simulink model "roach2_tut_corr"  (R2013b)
settings: Solver=VariableStepDiscrete  SolverMode=SingleTasking  StartTime=0.0  StopTime=100  RelTol=1e-3
undefined symbols (not defined in the file): add_latency, addr_width, Bit, bitfield, BitWidth, bram_latency, burst_size, casper_library_scopes, conv_latency, data_width, DelayLen, fan_latency, FFTSize, FFTStage, getfield, increment, led, Location, Lower, mult_latency, mux_latency, n_bits, n_bits_data, n_inputs, n_streams, n_taps, neg_latency, negate_latency, nsamples, pfb_size, pulse_len, reset_period, ROACH, ROACH2, snapshot, sx475t, sync_period, sync_period_bits, Upper, UseCounter, Width
libraries: xbsIndex_r4 x24444, casper_library_misc x73, xbsReplacements_r4 x34, casper_library_delays x14, xps_library x7
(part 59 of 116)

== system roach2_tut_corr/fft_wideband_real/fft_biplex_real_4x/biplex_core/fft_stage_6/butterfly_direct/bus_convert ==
  din : Inport
  bussify : Subsystem  AncestorBlock=casper_library_flow_control/bus_create
  conv1 : Subsystem  AncestorBlock=casper_library_misc/convert_of
  conv10 : Subsystem  AncestorBlock=casper_library_misc/convert_of
  conv11 : Subsystem  AncestorBlock=casper_library_misc/convert_of
  conv12 : Subsystem  AncestorBlock=casper_library_misc/convert_of
  conv13 : Subsystem  AncestorBlock=casper_library_misc/convert_of
  conv14 : Subsystem  AncestorBlock=casper_library_misc/convert_of
  conv15 : Subsystem  AncestorBlock=casper_library_misc/convert_of
  conv16 : Subsystem  AncestorBlock=casper_library_misc/convert_of
  conv2 : Subsystem  AncestorBlock=casper_library_misc/convert_of
  conv3 : Subsystem  AncestorBlock=casper_library_misc/convert_of
  conv4 : Subsystem  AncestorBlock=casper_library_misc/convert_of
  conv5 : Subsystem  AncestorBlock=casper_library_misc/convert_of
  conv6 : Subsystem  AncestorBlock=casper_library_misc/convert_of
  conv7 : Subsystem  AncestorBlock=casper_library_misc/convert_of
  conv8 : Subsystem  AncestorBlock=casper_library_misc/convert_of
  conv9 : Subsystem  AncestorBlock=casper_library_misc/convert_of
  debus : Subsystem  AncestorBlock=casper_library_flow_control/bus_expand
  of_bussify : Subsystem  AncestorBlock=casper_library_flow_control/bus_create
  dout : Outport
  overflow : Outport  Port=2
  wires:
  din/1 -> debus/1(bus_in)
  debus/1(msb_out16) -> conv1/1(din)
  debus/2(out15) -> conv2/1(din)
  debus/3(out14) -> conv3/1(din)
  debus/4(out13) -> conv4/1(din)
  debus/5(out12) -> conv5/1(din)
  debus/6(out11) -> conv6/1(din)
  debus/7(out10) -> conv7/1(din)
  debus/8(out9) -> conv8/1(din)
  debus/9(out8) -> conv9/1(din)
  debus/10(out7) -> conv10/1(din)
  debus/11(out6) -> conv11/1(din)
  debus/12(out5) -> conv12/1(din)
  debus/13(out4) -> conv13/1(din)
  debus/14(out3) -> conv14/1(din)
  debus/15(out2) -> conv15/1(din)
  debus/16(lsb_out1) -> conv16/1(din)
  conv1/1(dout) -> bussify/1(in1)
  conv2/1(dout) -> bussify/2(in2)
  conv3/1(dout) -> bussify/3(in3)
  conv4/1(dout) -> bussify/4(in4)
  conv5/1(dout) -> bussify/5(in5)
  conv6/1(dout) -> bussify/6(in6)
  conv7/1(dout) -> bussify/7(in7)
  conv8/1(dout) -> bussify/8(in8)
  conv9/1(dout) -> bussify/9(in9)
  conv10/1(dout) -> bussify/10(in10)
  conv11/1(dout) -> bussify/11(in11)
  conv12/1(dout) -> bussify/12(in12)
  conv13/1(dout) -> bussify/13(in13)
  conv14/1(dout) -> bussify/14(in14)
  conv15/1(dout) -> bussify/15(in15)
  conv16/1(dout) -> bussify/16(in16)
  conv1/2(of) -> of_bussify/1(in1)
  conv2/2(of) -> of_bussify/2(in2)
  conv3/2(of) -> of_bussify/3(in3)
  conv4/2(of) -> of_bussify/4(in4)
  conv5/2(of) -> of_bussify/5(in5)
  conv6/2(of) -> of_bussify/6(in6)
  conv7/2(of) -> of_bussify/7(in7)
  conv8/2(of) -> of_bussify/8(in8)
  conv9/2(of) -> of_bussify/9(in9)
  conv10/2(of) -> of_bussify/10(in10)
  conv11/2(of) -> of_bussify/11(in11)
  conv12/2(of) -> of_bussify/12(in12)
  conv13/2(of) -> of_bussify/13(in13)
  conv14/2(of) -> of_bussify/14(in14)
  conv15/2(of) -> of_bussify/15(in15)
  conv16/2(of) -> of_bussify/16(in16)
  bussify/1(bus_out) -> dout/1
  of_bussify/1(bus_out) -> overflow/1

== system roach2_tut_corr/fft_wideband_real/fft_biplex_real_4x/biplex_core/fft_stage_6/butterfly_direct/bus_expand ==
  bus_in : Inport
  reinterpret1 : xbsIndex_r4/Reinterpret  force_arith_type=on  arith_type=Unsigned  force_bin_pt=on  bin_pt=0  block_type=reinterpret
  reinterpret2 : xbsIndex_r4/Reinterpret  force_arith_type=on  arith_type=Unsigned  force_bin_pt=on  bin_pt=0  block_type=reinterpret
  slice1 : xbsIndex_r4/Slice  nbits=144  boolean_output=off  mode=Upper Bit Location + Width  bit1=-144  base1=MSB of Input  bit0=0  base0=LSB of Input  dbl_ovrd=off  block_type=slice
  slice2 : xbsIndex_r4/Slice  nbits=144  boolean_output=off  mode=Upper Bit Location + Width  bit1=0  base1=MSB of Input  bit0=0  base0=LSB of Input  dbl_ovrd=off  block_type=slice
  msb_out2 : Outport
  lsb_out1 : Outport  Port=2
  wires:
  bus_in/1 -> slice2/1, slice1/1
  slice2/1 -> reinterpret2/1
  reinterpret2/1 -> msb_out2/1
  slice1/1 -> reinterpret1/1
  reinterpret1/1 -> lsb_out1/1

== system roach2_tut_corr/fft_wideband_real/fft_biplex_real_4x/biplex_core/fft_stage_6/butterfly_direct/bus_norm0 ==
  din : Inport
  bussify : Subsystem  AncestorBlock=casper_library_flow_control/bus_create
  conv{1..16} (16 alike) : xbsIndex_r4/Convert  gui_display_data_type=Fixed-point  arith_type="Signed  (2's comp)"  n_bits=21  bin_pt=18  float_type=Single  exp_bits=8  fraction_bits=24  quantization=Truncate  overflow=Wrap  en=off  latency=0  dbl_ovrd=off  pipeline=on  block_type=convert
  debus : Subsystem  AncestorBlock=casper_library_flow_control/bus_expand
  dout : Outport
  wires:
  din/1 -> debus/1(bus_in)
  debus/1(msb_out16) -> conv1/1
  debus/2(out15) -> conv2/1
  debus/3(out14) -> conv3/1
  debus/4(out13) -> conv4/1
  debus/5(out12) -> conv5/1
  debus/6(out11) -> conv6/1
  debus/7(out10) -> conv7/1
  debus/8(out9) -> conv8/1
  debus/9(out8) -> conv9/1
  debus/10(out7) -> conv10/1
  debus/11(out6) -> conv11/1
  debus/12(out5) -> conv12/1
  debus/13(out4) -> conv13/1
  debus/14(out3) -> conv14/1
  debus/15(out2) -> conv15/1
  debus/16(lsb_out1) -> conv16/1
  conv1/1 -> bussify/1(in1)
  conv2/1 -> bussify/2(in2)
  conv3/1 -> bussify/3(in3)
  conv4/1 -> bussify/4(in4)
  conv5/1 -> bussify/5(in5)
  conv6/1 -> bussify/6(in6)
  conv7/1 -> bussify/7(in7)
  conv8/1 -> bussify/8(in8)
  conv9/1 -> bussify/9(in9)
  conv10/1 -> bussify/10(in10)
  conv11/1 -> bussify/11(in11)
  conv12/1 -> bussify/12(in12)
  conv13/1 -> bussify/13(in13)
  conv14/1 -> bussify/14(in14)
  conv15/1 -> bussify/15(in15)
  conv16/1 -> bussify/16(in16)
  bussify/1(bus_out) -> dout/1

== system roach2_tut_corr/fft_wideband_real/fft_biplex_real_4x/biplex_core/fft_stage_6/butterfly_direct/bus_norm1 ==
  din : Inport
  bussify : Subsystem  AncestorBlock=casper_library_flow_control/bus_create
  conv1 : Subsystem  AncestorBlock=casper_library_misc/convert
  conv10 : Subsystem  AncestorBlock=casper_library_misc/convert
  conv11 : Subsystem  AncestorBlock=casper_library_misc/convert
  conv12 : Subsystem  AncestorBlock=casper_library_misc/convert
  conv13 : Subsystem  AncestorBlock=casper_library_misc/convert
  conv14 : Subsystem  AncestorBlock=casper_library_misc/convert
  conv15 : Subsystem  AncestorBlock=casper_library_misc/convert
  conv16 : Subsystem  AncestorBlock=casper_library_misc/convert
  conv2 : Subsystem  AncestorBlock=casper_library_misc/convert
  conv3 : Subsystem  AncestorBlock=casper_library_misc/convert
  conv4 : Subsystem  AncestorBlock=casper_library_misc/convert
  conv5 : Subsystem  AncestorBlock=casper_library_misc/convert
  conv6 : Subsystem  AncestorBlock=casper_library_misc/convert
  conv7 : Subsystem  AncestorBlock=casper_library_misc/convert
  conv8 : Subsystem  AncestorBlock=casper_library_misc/convert
  conv9 : Subsystem  AncestorBlock=casper_library_misc/convert
  debus : Subsystem  AncestorBlock=casper_library_flow_control/bus_expand
  dout : Outport
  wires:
  din/1 -> debus/1(bus_in)
  debus/1(msb_out16) -> conv1/1(in)
  debus/2(out15) -> conv2/1(in)
  debus/3(out14) -> conv3/1(in)
  debus/4(out13) -> conv4/1(in)
  debus/5(out12) -> conv5/1(in)
  debus/6(out11) -> conv6/1(in)
  debus/7(out10) -> conv7/1(in)
  debus/8(out9) -> conv8/1(in)
  debus/9(out8) -> conv9/1(in)
  debus/10(out7) -> conv10/1(in)
  debus/11(out6) -> conv11/1(in)
  debus/12(out5) -> conv12/1(in)
  debus/13(out4) -> conv13/1(in)
  debus/14(out3) -> conv14/1(in)
  debus/15(out2) -> conv15/1(in)
  debus/16(lsb_out1) -> conv16/1(in)
  conv1/1(out) -> bussify/1(in1)
  conv2/1(out) -> bussify/2(in2)
  conv3/1(out) -> bussify/3(in3)
  conv4/1(out) -> bussify/4(in4)
  conv5/1(out) -> bussify/5(in5)
  conv6/1(out) -> bussify/6(in6)
  conv7/1(out) -> bussify/7(in7)
  conv8/1(out) -> bussify/8(in8)
  conv9/1(out) -> bussify/9(in9)
  conv10/1(out) -> bussify/10(in10)
  conv11/1(out) -> bussify/11(in11)
  conv12/1(out) -> bussify/12(in12)
  conv13/1(out) -> bussify/13(in13)
  conv14/1(out) -> bussify/14(in14)
  conv15/1(out) -> bussify/15(in15)
  conv16/1(out) -> bussify/16(in16)
  bussify/1(bus_out) -> dout/1

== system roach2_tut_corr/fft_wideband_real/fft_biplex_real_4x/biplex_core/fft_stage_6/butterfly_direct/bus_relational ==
  a : Inport
  b : Inport  Port=2
  a_debus : Subsystem  AncestorBlock=casper_library_flow_control/bus_expand
  b_debus : Subsystem  AncestorBlock=casper_library_flow_control/bus_expand
  bussify : Subsystem  AncestorBlock=casper_library_flow_control/bus_create
  relational{1..4} (4 alike) : xbsIndex_r4/Relational  mode=a!=b  en=off  latency=1  dbl_ovrd=off  block_type=relational
  a!=b : Outport
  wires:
  a/1 -> a_debus/1(bus_in)
  b/1 -> b_debus/1(bus_in)
  a_debus/1(msb_lsb_out1) -> relational1/1, relational2/1, relational3/1, relational4/1
  b_debus/1(msb_out4) -> relational1/2
  b_debus/2(out3) -> relational2/2
  b_debus/3(out2) -> relational3/2
  b_debus/4(lsb_out1) -> relational4/2
  relational1/1 -> bussify/1(in1)
  relational2/1 -> bussify/2(in2)
  relational3/1 -> bussify/3(in3)
  relational4/1 -> bussify/4(in4)
  bussify/1(bus_out) -> a!=b/1

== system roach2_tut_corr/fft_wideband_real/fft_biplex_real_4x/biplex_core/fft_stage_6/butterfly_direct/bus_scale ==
  din : Inport
  bussify : Subsystem  AncestorBlock=casper_library_flow_control/bus_create
  debus : Subsystem  AncestorBlock=casper_library_flow_control/bus_expand
  scale{1..16} (16 alike) : xbsIndex_r4/Scale  scale_factor=-1  dbl_ovrd=off  block_type=scale
  dout : Outport
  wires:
  din/1 -> debus/1(bus_in)
  debus/1(msb_out16) -> scale1/1
  debus/2(out15) -> scale2/1
  debus/3(out14) -> scale3/1
  debus/4(out13) -> scale4/1
  debus/5(out12) -> scale5/1
  debus/6(out11) -> scale6/1
  debus/7(out10) -> scale7/1
  debus/8(out9) -> scale8/1
  debus/9(out8) -> scale9/1
  debus/10(out7) -> scale10/1
  debus/11(out6) -> scale11/1
  debus/12(out5) -> scale12/1
  debus/13(out4) -> scale13/1
  debus/14(out3) -> scale14/1
  debus/15(out2) -> scale15/1
  debus/16(lsb_out1) -> scale16/1
  scale1/1 -> bussify/1(in1)
  scale2/1 -> bussify/2(in2)
  scale3/1 -> bussify/3(in3)
  scale4/1 -> bussify/4(in4)
  scale5/1 -> bussify/5(in5)
  scale6/1 -> bussify/6(in6)
  scale7/1 -> bussify/7(in7)
  scale8/1 -> bussify/8(in8)
  scale9/1 -> bussify/9(in9)
  scale10/1 -> bussify/10(in10)
  scale11/1 -> bussify/11(in11)
  scale12/1 -> bussify/12(in12)
  scale13/1 -> bussify/13(in13)
  scale14/1 -> bussify/14(in14)
  scale15/1 -> bussify/15(in15)
  scale16/1 -> bussify/16(in16)
  bussify/1(bus_out) -> dout/1

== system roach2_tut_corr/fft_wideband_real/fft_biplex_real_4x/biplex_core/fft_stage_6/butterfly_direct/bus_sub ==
  a : Inport
  b : Inport  Port=2
  a_debus : Subsystem  AncestorBlock=casper_library_flow_control/bus_expand
  addsub{1..8} (8 alike) : xbsIndex_r4/AddSub  mode=Subtraction  use_carryin=off  use_carryout=off  en=off  latency=1  precision=User Defined  arith_type="Signed  (2's comp)"  n_bits=20  bin_pt=17  quantization=Truncate  overflow=Wrap  dbl_ovrd=off  use_behavioral_HDL=on  hw_selection=Fabric  pipelined=on  block_type=addsub
  b_debus : Subsystem  AncestorBlock=casper_library_flow_control/bus_expand
  op_bussify : Subsystem  AncestorBlock=casper_library_flow_control/bus_create
  dout : Outport
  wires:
  a/1 -> a_debus/1(bus_in)
  b/1 -> b_debus/1(bus_in)
  a_debus/1(msb_out8) -> addsub1/1
  b_debus/1(msb_out8) -> addsub1/2
  a_debus/2(out7) -> addsub2/1
  b_debus/2(out7) -> addsub2/2
  a_debus/3(out6) -> addsub3/1
  b_debus/3(out6) -> addsub3/2
  a_debus/4(out5) -> addsub4/1
  b_debus/4(out5) -> addsub4/2
  a_debus/5(out4) -> addsub5/1
  b_debus/5(out4) -> addsub5/2
  a_debus/6(out3) -> addsub6/1
  b_debus/6(out3) -> addsub6/2
  a_debus/7(out2) -> addsub7/1
  b_debus/7(out2) -> addsub7/2
  a_debus/8(lsb_out1) -> addsub8/1
  b_debus/8(lsb_out1) -> addsub8/2
  addsub1/1 -> op_bussify/1(in1)
  addsub2/1 -> op_bussify/2(in2)
  addsub3/1 -> op_bussify/3(in3)
  addsub4/1 -> op_bussify/4(in4)
  addsub5/1 -> op_bussify/5(in5)
  addsub6/1 -> op_bussify/6(in6)
  addsub7/1 -> op_bussify/7(in7)
  addsub8/1 -> op_bussify/8(in8)
  op_bussify/1(bus_out) -> dout/1

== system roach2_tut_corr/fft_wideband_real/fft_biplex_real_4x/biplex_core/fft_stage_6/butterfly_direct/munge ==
  din : Inport
  join : Subsystem  AncestorBlock=casper_library_flow_control/bus_create
  reinterpret : xbsIndex_r4/Reinterpret  force_arith_type=on  arith_type=Unsigned  force_bin_pt=on  bin_pt=0  block_type=reinterpret
  reinterpret_out : xbsIndex_r4/Reinterpret  force_arith_type=on  arith_type=Unsigned  force_bin_pt=on  bin_pt=0  block_type=reinterpret
  split : Subsystem  AncestorBlock=casper_library_flow_control/bus_expand
  dout : Outport
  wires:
  reinterpret_out/1 -> dout/1
  din/1 -> reinterpret/1
  reinterpret/1 -> split/1(bus_in)
  join/1(bus_out) -> reinterpret_out/1
  split/1(msb_out8) -> join/1(in1)
  split/5(out4) -> join/2(in2)
  split/2(out7) -> join/3(in3)
  split/6(out3) -> join/4(in4)
  split/3(out6) -> join/5(in5)
  split/7(out2) -> join/6(in6)
  split/4(out5) -> join/7(in7)
  split/8(lsb_out1) -> join/8(in8)

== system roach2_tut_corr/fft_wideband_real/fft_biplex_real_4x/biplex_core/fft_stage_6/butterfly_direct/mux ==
  sel : Inport
  d0 : Inport  Port=2
  d1 : Inport  Port=3
  d_bussify : Subsystem  AncestorBlock=casper_library_flow_control/bus_create
  expand0 : Subsystem  AncestorBlock=casper_library_flow_control/bus_expand
  expand1 : Subsystem  AncestorBlock=casper_library_flow_control/bus_expand
  mux{0..15} (16 alike) : xbsIndex_r4/Mux  inputs=2  en=off  latency=2  precision=Full  arith_type=Unsigned  n_bits=16  bin_pt=14  quantization=Truncate  overflow=Wrap  dbl_ovrd=off  block_type=mux
  sel_expand : Subsystem  AncestorBlock=casper_library_flow_control/bus_expand
  out : Outport
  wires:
  sel/1 -> sel_expand/1(bus_in)
  d0/1 -> expand0/1(bus_in)
  d1/1 -> expand1/1(bus_in)
  sel_expand/1(msb_out16) -> mux0/1
  expand0/1(msb_out16) -> mux0/2
  expand1/1(msb_out16) -> mux0/3
  sel_expand/2(out15) -> mux1/1
  expand0/2(out15) -> mux1/2
  expand1/2(out15) -> mux1/3
  sel_expand/3(out14) -> mux2/1
  expand0/3(out14) -> mux2/2
  expand1/3(out14) -> mux2/3
  sel_expand/4(out13) -> mux3/1
  expand0/4(out13) -> mux3/2
  expand1/4(out13) -> mux3/3
  sel_expand/5(out12) -> mux4/1
  expand0/5(out12) -> mux4/2
  expand1/5(out12) -> mux4/3
  sel_expand/6(out11) -> mux5/1
  expand0/6(out11) -> mux5/2
  expand1/6(out11) -> mux5/3
  sel_expand/7(out10) -> mux6/1
  expand0/7(out10) -> mux6/2
  expand1/7(out10) -> mux6/3
  sel_expand/8(out9) -> mux7/1
  expand0/8(out9) -> mux7/2
  expand1/8(out9) -> mux7/3
  sel_expand/9(out8) -> mux8/1
  expand0/9(out8) -> mux8/2
  expand1/9(out8) -> mux8/3
  sel_expand/10(out7) -> mux9/1
  expand0/10(out7) -> mux9/2
  expand1/10(out7) -> mux9/3
  sel_expand/11(out6) -> mux10/1
  expand0/11(out6) -> mux10/2
  expand1/11(out6) -> mux10/3
  sel_expand/12(out5) -> mux11/1
  expand0/12(out5) -> mux11/2
  expand1/12(out5) -> mux11/3
  sel_expand/13(out4) -> mux12/1
  expand0/13(out4) -> mux12/2
  expand1/13(out4) -> mux12/3
  sel_expand/14(out3) -> mux13/1
  expand0/14(out3) -> mux13/2
  expand1/14(out3) -> mux13/3
  sel_expand/15(out2) -> mux14/1
  expand0/15(out2) -> mux14/2
  expand1/15(out2) -> mux14/3
  sel_expand/16(lsb_out1) -> mux15/1
  expand0/16(lsb_out1) -> mux15/2
  expand1/16(lsb_out1) -> mux15/3
  mux0/1 -> d_bussify/1(in1)
  mux1/1 -> d_bussify/2(in2)
  mux2/1 -> d_bussify/3(in3)
  mux3/1 -> d_bussify/4(in4)
  mux4/1 -> d_bussify/5(in5)
  mux5/1 -> d_bussify/6(in6)
  mux6/1 -> d_bussify/7(in7)
  mux7/1 -> d_bussify/8(in8)
  mux8/1 -> d_bussify/9(in9)
  mux9/1 -> d_bussify/10(in10)
  mux10/1 -> d_bussify/11(in11)
  mux11/1 -> d_bussify/12(in12)
  mux12/1 -> d_bussify/13(in13)
  mux13/1 -> d_bussify/14(in14)
  mux14/1 -> d_bussify/15(in15)
  mux15/1 -> d_bussify/16(in16)
  d_bussify/1(bus_out) -> out/1

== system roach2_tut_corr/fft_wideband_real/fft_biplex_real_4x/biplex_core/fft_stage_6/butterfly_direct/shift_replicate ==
  in : Inport
  bussify : Subsystem  AncestorBlock=casper_library_flow_control/bus_create
  din0_{0..15} (16 alike) : xbsIndex_r4/Delay  rst=off  infoeditControl=Selection of Reset will increase slice count due to use of real FFs and instead of SRLs  en=off  latency=1  dbl_ovrd=off  reg_retiming=off  block_type=delay
  out : Outport
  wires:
  in/1 -> din0_0/1, din0_1/1, din0_2/1, din0_3/1, din0_4/1, din0_5/1, din0_6/1, din0_7/1, din0_8/1, din0_9/1, din0_10/1, din0_11/1, din0_12/1, din0_13/1, din0_14/1, din0_15/1
  din0_0/1 -> bussify/1(in1)
  din0_1/1 -> bussify/2(in2)
  din0_2/1 -> bussify/3(in3)
  din0_3/1 -> bussify/4(in4)
  din0_4/1 -> bussify/5(in5)
  din0_5/1 -> bussify/6(in6)
  din0_6/1 -> bussify/7(in7)
  din0_7/1 -> bussify/8(in8)
  din0_8/1 -> bussify/9(in9)
  din0_9/1 -> bussify/10(in10)
  din0_10/1 -> bussify/11(in11)
  din0_11/1 -> bussify/12(in12)
  din0_12/1 -> bussify/13(in13)
  din0_13/1 -> bussify/14(in14)
  din0_14/1 -> bussify/15(in15)
  din0_15/1 -> bussify/16(in16)
  bussify/1(bus_out) -> out/1

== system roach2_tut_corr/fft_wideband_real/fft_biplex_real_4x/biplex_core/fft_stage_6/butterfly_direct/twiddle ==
  ai : Inport
  bi : Inport  Port=2
  sync_in : Inport  Port=3
  bus_convert : Subsystem  AncestorBlock=casper_library_bus/bus_convert
  bus_create : Subsystem  AncestorBlock=casper_library_flow_control/bus_create
  bus_expand : Subsystem  AncestorBlock=casper_library_flow_control/bus_expand
  bus_expand1 : Subsystem  AncestorBlock=casper_library_flow_control/bus_expand
  bus_mult : Subsystem  AncestorBlock=casper_library_bus/bus_mult
  coeff_gen : Subsystem  AncestorBlock=casper_library_ffts_twiddle_coeff_gen/coeff_gen
  ao : Outport
  bwo : Outport  Port=2
  sync_out : Outport  Port=3
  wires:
  bi/1 -> bus_create/1(in1)
  sync_in/1 -> bus_create/2(in2), coeff_gen/1(rst)
  ai/1 -> bus_create/3(in3)
  bus_create/1(bus_out) -> coeff_gen/2(misci)
  coeff_gen/2(misco) -> bus_expand/1(bus_in)
  coeff_gen/1(w) -> bus_mult/1(a)
  bus_expand/2(lsb_out1) -> bus_mult/3(misci)
  bus_expand/1(msb_out2) -> bus_mult/2(b)
  bus_mult/1(a*b) -> bus_convert/1(din)
  bus_mult/2(misco) -> bus_convert/2(misci)
  bus_convert/1(dout) -> bwo/1
  bus_convert/2(misco) -> bus_expand1/1(bus_in)
  bus_expand1/1(msb_out2) -> sync_out/1
  bus_expand1/2(lsb_out1) -> ao/1

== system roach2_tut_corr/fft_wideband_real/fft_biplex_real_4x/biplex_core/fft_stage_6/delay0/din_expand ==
  bus_in : Inport
  reinterpret{1..4} (4 alike) : xbsIndex_r4/Reinterpret  force_arith_type=on  arith_type=Unsigned  force_bin_pt=on  bin_pt=0  block_type=reinterpret
  slice1 : xbsIndex_r4/Slice  nbits=36  boolean_output=off  mode=Upper Bit Location + Width  bit1=-108  base1=MSB of Input  bit0=0  base0=LSB of Input  dbl_ovrd=off  block_type=slice
  slice2 : xbsIndex_r4/Slice  nbits=36  boolean_output=off  mode=Upper Bit Location + Width  bit1=-72  base1=MSB of Input  bit0=0  base0=LSB of Input  dbl_ovrd=off  block_type=slice
  slice3 : xbsIndex_r4/Slice  nbits=36  boolean_output=off  mode=Upper Bit Location + Width  bit1=-36  base1=MSB of Input  bit0=0  base0=LSB of Input  dbl_ovrd=off  block_type=slice
  slice4 : xbsIndex_r4/Slice  nbits=36  boolean_output=off  mode=Upper Bit Location + Width  bit1=0  base1=MSB of Input  bit0=0  base0=LSB of Input  dbl_ovrd=off  block_type=slice
  msb_out4 : Outport
  out3 : Outport  Port=2
  out2 : Outport  Port=3
  lsb_out1 : Outport  Port=4
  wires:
  bus_in/1 -> slice4/1, slice3/1, slice2/1, slice1/1
  slice4/1 -> reinterpret4/1
  reinterpret4/1 -> msb_out4/1
  slice3/1 -> reinterpret3/1
  reinterpret3/1 -> out3/1
  slice2/1 -> reinterpret2/1
  reinterpret2/1 -> out2/1
  slice1/1 -> reinterpret1/1
  reinterpret1/1 -> lsb_out1/1

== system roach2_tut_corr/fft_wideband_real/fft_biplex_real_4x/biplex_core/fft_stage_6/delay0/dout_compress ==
  in1 : Inport
  in2 : Inport  Port=2
  in3 : Inport  Port=3
  in4 : Inport  Port=4
  concatenate : xbsIndex_r4/Concat  num_inputs=4  dbl_ovrd=off  block_type=concat
  reinterpret{1..4} (4 alike) : xbsIndex_r4/Reinterpret  force_arith_type=on  arith_type=Unsigned  force_bin_pt=on  bin_pt=0  block_type=reinterpret
  bus_out : Outport
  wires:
  concatenate/1 -> bus_out/1
  in1/1 -> reinterpret1/1
  reinterpret1/1 -> concatenate/1
  in2/1 -> reinterpret2/1
  reinterpret2/1 -> concatenate/2
  in3/1 -> reinterpret3/1
  reinterpret3/1 -> concatenate/3
  in4/1 -> reinterpret4/1
  reinterpret4/1 -> concatenate/4

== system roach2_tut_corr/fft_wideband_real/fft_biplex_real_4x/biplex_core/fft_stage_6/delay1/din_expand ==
  bus_in : Inport
  reinterpret{1..4} (4 alike) : xbsIndex_r4/Reinterpret  force_arith_type=on  arith_type=Unsigned  force_bin_pt=on  bin_pt=0  block_type=reinterpret
  slice1 : xbsIndex_r4/Slice  nbits=36  boolean_output=off  mode=Upper Bit Location + Width  bit1=-108  base1=MSB of Input  bit0=0  base0=LSB of Input  dbl_ovrd=off  block_type=slice
  slice2 : xbsIndex_r4/Slice  nbits=36  boolean_output=off  mode=Upper Bit Location + Width  bit1=-72  base1=MSB of Input  bit0=0  base0=LSB of Input  dbl_ovrd=off  block_type=slice
  slice3 : xbsIndex_r4/Slice  nbits=36  boolean_output=off  mode=Upper Bit Location + Width  bit1=-36  base1=MSB of Input  bit0=0  base0=LSB of Input  dbl_ovrd=off  block_type=slice
  slice4 : xbsIndex_r4/Slice  nbits=36  boolean_output=off  mode=Upper Bit Location + Width  bit1=0  base1=MSB of Input  bit0=0  base0=LSB of Input  dbl_ovrd=off  block_type=slice
  msb_out4 : Outport
  out3 : Outport  Port=2
  out2 : Outport  Port=3
  lsb_out1 : Outport  Port=4
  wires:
  bus_in/1 -> slice4/1, slice3/1, slice2/1, slice1/1
  slice4/1 -> reinterpret4/1
  reinterpret4/1 -> msb_out4/1
  slice3/1 -> reinterpret3/1
  reinterpret3/1 -> out3/1
  slice2/1 -> reinterpret2/1
  reinterpret2/1 -> out2/1
  slice1/1 -> reinterpret1/1
  reinterpret1/1 -> lsb_out1/1

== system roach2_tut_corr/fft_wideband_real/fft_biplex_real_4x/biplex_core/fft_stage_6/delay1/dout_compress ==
  in1 : Inport
  in2 : Inport  Port=2
  in3 : Inport  Port=3
  in4 : Inport  Port=4
  concatenate : xbsIndex_r4/Concat  num_inputs=4  dbl_ovrd=off  block_type=concat
  reinterpret{1..4} (4 alike) : xbsIndex_r4/Reinterpret  force_arith_type=on  arith_type=Unsigned  force_bin_pt=on  bin_pt=0  block_type=reinterpret
  bus_out : Outport
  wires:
  concatenate/1 -> bus_out/1
  in1/1 -> reinterpret1/1
  reinterpret1/1 -> concatenate/1
  in2/1 -> reinterpret2/1
  reinterpret2/1 -> concatenate/2
  in3/1 -> reinterpret3/1
  reinterpret3/1 -> concatenate/3
  in4/1 -> reinterpret4/1
  reinterpret4/1 -> concatenate/4

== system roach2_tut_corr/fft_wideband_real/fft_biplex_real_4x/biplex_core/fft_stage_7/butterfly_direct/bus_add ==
  a : Inport
  b : Inport  Port=2
  a_debus : Subsystem  AncestorBlock=casper_library_flow_control/bus_expand
  addsub{1..8} (8 alike) : xbsIndex_r4/AddSub  mode=Addition  use_carryin=off  use_carryout=off  en=off  latency=1  precision=User Defined  arith_type="Signed  (2's comp)"  n_bits=20  bin_pt=17  quantization=Truncate  overflow=Wrap  dbl_ovrd=off  use_behavioral_HDL=on  hw_selection=Fabric  pipelined=on  block_type=addsub
  b_debus : Subsystem  AncestorBlock=casper_library_flow_control/bus_expand
  op_bussify : Subsystem  AncestorBlock=casper_library_flow_control/bus_create
  dout : Outport
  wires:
  a/1 -> a_debus/1(bus_in)
  b/1 -> b_debus/1(bus_in)
  a_debus/1(msb_out8) -> addsub1/1
  b_debus/1(msb_out8) -> addsub1/2
  a_debus/2(out7) -> addsub2/1
  b_debus/2(out7) -> addsub2/2
  a_debus/3(out6) -> addsub3/1
  b_debus/3(out6) -> addsub3/2
  a_debus/4(out5) -> addsub4/1
  b_debus/4(out5) -> addsub4/2
  a_debus/5(out4) -> addsub5/1
  b_debus/5(out4) -> addsub5/2
  a_debus/6(out3) -> addsub6/1
  b_debus/6(out3) -> addsub6/2
  a_debus/7(out2) -> addsub7/1
  b_debus/7(out2) -> addsub7/2
  a_debus/8(lsb_out1) -> addsub8/1
  b_debus/8(lsb_out1) -> addsub8/2
  addsub1/1 -> op_bussify/1(in1)
  addsub2/1 -> op_bussify/2(in2)
  addsub3/1 -> op_bussify/3(in3)
  addsub4/1 -> op_bussify/4(in4)
  addsub5/1 -> op_bussify/5(in5)
  addsub6/1 -> op_bussify/6(in6)
  addsub7/1 -> op_bussify/7(in7)
  addsub8/1 -> op_bussify/8(in8)
  op_bussify/1(bus_out) -> dout/1

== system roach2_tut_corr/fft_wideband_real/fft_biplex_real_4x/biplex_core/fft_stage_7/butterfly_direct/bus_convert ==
  din : Inport
  bussify : Subsystem  AncestorBlock=casper_library_flow_control/bus_create
  conv1 : Subsystem  AncestorBlock=casper_library_misc/convert_of
  conv10 : Subsystem  AncestorBlock=casper_library_misc/convert_of
  conv11 : Subsystem  AncestorBlock=casper_library_misc/convert_of
  conv12 : Subsystem  AncestorBlock=casper_library_misc/convert_of
  conv13 : Subsystem  AncestorBlock=casper_library_misc/convert_of
  conv14 : Subsystem  AncestorBlock=casper_library_misc/convert_of
  conv15 : Subsystem  AncestorBlock=casper_library_misc/convert_of
  conv16 : Subsystem  AncestorBlock=casper_library_misc/convert_of
  conv2 : Subsystem  AncestorBlock=casper_library_misc/convert_of
  conv3 : Subsystem  AncestorBlock=casper_library_misc/convert_of
  conv4 : Subsystem  AncestorBlock=casper_library_misc/convert_of
  conv5 : Subsystem  AncestorBlock=casper_library_misc/convert_of
  conv6 : Subsystem  AncestorBlock=casper_library_misc/convert_of
  conv7 : Subsystem  AncestorBlock=casper_library_misc/convert_of
  conv8 : Subsystem  AncestorBlock=casper_library_misc/convert_of
  conv9 : Subsystem  AncestorBlock=casper_library_misc/convert_of
  debus : Subsystem  AncestorBlock=casper_library_flow_control/bus_expand
  of_bussify : Subsystem  AncestorBlock=casper_library_flow_control/bus_create
  dout : Outport
  overflow : Outport  Port=2
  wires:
  din/1 -> debus/1(bus_in)
  debus/1(msb_out16) -> conv1/1(din)
  debus/2(out15) -> conv2/1(din)
  debus/3(out14) -> conv3/1(din)
  debus/4(out13) -> conv4/1(din)
  debus/5(out12) -> conv5/1(din)
  debus/6(out11) -> conv6/1(din)
  debus/7(out10) -> conv7/1(din)
  debus/8(out9) -> conv8/1(din)
  debus/9(out8) -> conv9/1(din)
  debus/10(out7) -> conv10/1(din)
  debus/11(out6) -> conv11/1(din)
  debus/12(out5) -> conv12/1(din)
  debus/13(out4) -> conv13/1(din)
  debus/14(out3) -> conv14/1(din)
  debus/15(out2) -> conv15/1(din)
  debus/16(lsb_out1) -> conv16/1(din)
  conv1/1(dout) -> bussify/1(in1)
  conv2/1(dout) -> bussify/2(in2)
  conv3/1(dout) -> bussify/3(in3)
  conv4/1(dout) -> bussify/4(in4)
  conv5/1(dout) -> bussify/5(in5)
  conv6/1(dout) -> bussify/6(in6)
  conv7/1(dout) -> bussify/7(in7)
  conv8/1(dout) -> bussify/8(in8)
  conv9/1(dout) -> bussify/9(in9)
  conv10/1(dout) -> bussify/10(in10)
  conv11/1(dout) -> bussify/11(in11)
  conv12/1(dout) -> bussify/12(in12)
  conv13/1(dout) -> bussify/13(in13)
  conv14/1(dout) -> bussify/14(in14)
  conv15/1(dout) -> bussify/15(in15)
  conv16/1(dout) -> bussify/16(in16)
  conv1/2(of) -> of_bussify/1(in1)
  conv2/2(of) -> of_bussify/2(in2)
  conv3/2(of) -> of_bussify/3(in3)
  conv4/2(of) -> of_bussify/4(in4)
  conv5/2(of) -> of_bussify/5(in5)
  conv6/2(of) -> of_bussify/6(in6)
  conv7/2(of) -> of_bussify/7(in7)
  conv8/2(of) -> of_bussify/8(in8)
  conv9/2(of) -> of_bussify/9(in9)
  conv10/2(of) -> of_bussify/10(in10)
  conv11/2(of) -> of_bussify/11(in11)
  conv12/2(of) -> of_bussify/12(in12)
  conv13/2(of) -> of_bussify/13(in13)
  conv14/2(of) -> of_bussify/14(in14)
  conv15/2(of) -> of_bussify/15(in15)
  conv16/2(of) -> of_bussify/16(in16)
  bussify/1(bus_out) -> dout/1
  of_bussify/1(bus_out) -> overflow/1

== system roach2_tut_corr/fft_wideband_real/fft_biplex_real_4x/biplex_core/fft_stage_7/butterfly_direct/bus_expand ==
  bus_in : Inport
  reinterpret1 : xbsIndex_r4/Reinterpret  force_arith_type=on  arith_type=Unsigned  force_bin_pt=on  bin_pt=0  block_type=reinterpret
  reinterpret2 : xbsIndex_r4/Reinterpret  force_arith_type=on  arith_type=Unsigned  force_bin_pt=on  bin_pt=0  block_type=reinterpret
  slice1 : xbsIndex_r4/Slice  nbits=144  boolean_output=off  mode=Upper Bit Location + Width  bit1=-144  base1=MSB of Input  bit0=0  base0=LSB of Input  dbl_ovrd=off  block_type=slice
  slice2 : xbsIndex_r4/Slice  nbits=144  boolean_output=off  mode=Upper Bit Location + Width  bit1=0  base1=MSB of Input  bit0=0  base0=LSB of Input  dbl_ovrd=off  block_type=slice
  msb_out2 : Outport
  lsb_out1 : Outport  Port=2
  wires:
  bus_in/1 -> slice2/1, slice1/1
  slice2/1 -> reinterpret2/1
  reinterpret2/1 -> msb_out2/1
  slice1/1 -> reinterpret1/1
  reinterpret1/1 -> lsb_out1/1

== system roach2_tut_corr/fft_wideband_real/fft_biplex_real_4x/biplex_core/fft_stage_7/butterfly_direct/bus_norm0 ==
  din : Inport
  bussify : Subsystem  AncestorBlock=casper_library_flow_control/bus_create
  conv{1..16} (16 alike) : xbsIndex_r4/Convert  gui_display_data_type=Fixed-point  arith_type="Signed  (2's comp)"  n_bits=21  bin_pt=18  float_type=Single  exp_bits=8  fraction_bits=24  quantization=Truncate  overflow=Wrap  en=off  latency=0  dbl_ovrd=off  pipeline=on  block_type=convert
  debus : Subsystem  AncestorBlock=casper_library_flow_control/bus_expand
  dout : Outport
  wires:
  din/1 -> debus/1(bus_in)
  debus/1(msb_out16) -> conv1/1
  debus/2(out15) -> conv2/1
  debus/3(out14) -> conv3/1
  debus/4(out13) -> conv4/1
  debus/5(out12) -> conv5/1
  debus/6(out11) -> conv6/1
  debus/7(out10) -> conv7/1
  debus/8(out9) -> conv8/1
  debus/9(out8) -> conv9/1
  debus/10(out7) -> conv10/1
  debus/11(out6) -> conv11/1
  debus/12(out5) -> conv12/1
  debus/13(out4) -> conv13/1
  debus/14(out3) -> conv14/1
  debus/15(out2) -> conv15/1
  debus/16(lsb_out1) -> conv16/1
  conv1/1 -> bussify/1(in1)
  conv2/1 -> bussify/2(in2)
  conv3/1 -> bussify/3(in3)
  conv4/1 -> bussify/4(in4)
  conv5/1 -> bussify/5(in5)
  conv6/1 -> bussify/6(in6)
  conv7/1 -> bussify/7(in7)
  conv8/1 -> bussify/8(in8)
  conv9/1 -> bussify/9(in9)
  conv10/1 -> bussify/10(in10)
  conv11/1 -> bussify/11(in11)
  conv12/1 -> bussify/12(in12)
  conv13/1 -> bussify/13(in13)
  conv14/1 -> bussify/14(in14)
  conv15/1 -> bussify/15(in15)
  conv16/1 -> bussify/16(in16)
  bussify/1(bus_out) -> dout/1

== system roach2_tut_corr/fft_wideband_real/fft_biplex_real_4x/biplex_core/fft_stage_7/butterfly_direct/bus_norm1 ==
  din : Inport
  bussify : Subsystem  AncestorBlock=casper_library_flow_control/bus_create
  conv1 : Subsystem  AncestorBlock=casper_library_misc/convert
  conv10 : Subsystem  AncestorBlock=casper_library_misc/convert
  conv11 : Subsystem  AncestorBlock=casper_library_misc/convert
  conv12 : Subsystem  AncestorBlock=casper_library_misc/convert
  conv13 : Subsystem  AncestorBlock=casper_library_misc/convert
  conv14 : Subsystem  AncestorBlock=casper_library_misc/convert
  conv15 : Subsystem  AncestorBlock=casper_library_misc/convert
  conv16 : Subsystem  AncestorBlock=casper_library_misc/convert
  conv2 : Subsystem  AncestorBlock=casper_library_misc/convert
  conv3 : Subsystem  AncestorBlock=casper_library_misc/convert
  conv4 : Subsystem  AncestorBlock=casper_library_misc/convert
  conv5 : Subsystem  AncestorBlock=casper_library_misc/convert
  conv6 : Subsystem  AncestorBlock=casper_library_misc/convert
  conv7 : Subsystem  AncestorBlock=casper_library_misc/convert
  conv8 : Subsystem  AncestorBlock=casper_library_misc/convert
  conv9 : Subsystem  AncestorBlock=casper_library_misc/convert
  debus : Subsystem  AncestorBlock=casper_library_flow_control/bus_expand
  dout : Outport
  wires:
  din/1 -> debus/1(bus_in)
  debus/1(msb_out16) -> conv1/1(in)
  debus/2(out15) -> conv2/1(in)
  debus/3(out14) -> conv3/1(in)
  debus/4(out13) -> conv4/1(in)
  debus/5(out12) -> conv5/1(in)
  debus/6(out11) -> conv6/1(in)
  debus/7(out10) -> conv7/1(in)
  debus/8(out9) -> conv8/1(in)
  debus/9(out8) -> conv9/1(in)
  debus/10(out7) -> conv10/1(in)
  debus/11(out6) -> conv11/1(in)
  debus/12(out5) -> conv12/1(in)
  debus/13(out4) -> conv13/1(in)
  debus/14(out3) -> conv14/1(in)
  debus/15(out2) -> conv15/1(in)
  debus/16(lsb_out1) -> conv16/1(in)
  conv1/1(out) -> bussify/1(in1)
  conv2/1(out) -> bussify/2(in2)
  conv3/1(out) -> bussify/3(in3)
  conv4/1(out) -> bussify/4(in4)
  conv5/1(out) -> bussify/5(in5)
  conv6/1(out) -> bussify/6(in6)
  conv7/1(out) -> bussify/7(in7)
  conv8/1(out) -> bussify/8(in8)
  conv9/1(out) -> bussify/9(in9)
  conv10/1(out) -> bussify/10(in10)
  conv11/1(out) -> bussify/11(in11)
  conv12/1(out) -> bussify/12(in12)
  conv13/1(out) -> bussify/13(in13)
  conv14/1(out) -> bussify/14(in14)
  conv15/1(out) -> bussify/15(in15)
  conv16/1(out) -> bussify/16(in16)
  bussify/1(bus_out) -> dout/1

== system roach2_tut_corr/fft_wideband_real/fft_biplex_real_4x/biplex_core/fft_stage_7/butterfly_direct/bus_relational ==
  a : Inport
  b : Inport  Port=2
  a_debus : Subsystem  AncestorBlock=casper_library_flow_control/bus_expand
  b_debus : Subsystem  AncestorBlock=casper_library_flow_control/bus_expand
  bussify : Subsystem  AncestorBlock=casper_library_flow_control/bus_create
  relational{1..4} (4 alike) : xbsIndex_r4/Relational  mode=a!=b  en=off  latency=1  dbl_ovrd=off  block_type=relational
  a!=b : Outport
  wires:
  a/1 -> a_debus/1(bus_in)
  b/1 -> b_debus/1(bus_in)
  a_debus/1(msb_lsb_out1) -> relational1/1, relational2/1, relational3/1, relational4/1
  b_debus/1(msb_out4) -> relational1/2
  b_debus/2(out3) -> relational2/2
  b_debus/3(out2) -> relational3/2
  b_debus/4(lsb_out1) -> relational4/2
  relational1/1 -> bussify/1(in1)
  relational2/1 -> bussify/2(in2)
  relational3/1 -> bussify/3(in3)
  relational4/1 -> bussify/4(in4)
  bussify/1(bus_out) -> a!=b/1

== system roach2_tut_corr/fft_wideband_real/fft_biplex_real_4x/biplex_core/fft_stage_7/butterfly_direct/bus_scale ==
  din : Inport
  bussify : Subsystem  AncestorBlock=casper_library_flow_control/bus_create
  debus : Subsystem  AncestorBlock=casper_library_flow_control/bus_expand
  scale{1..16} (16 alike) : xbsIndex_r4/Scale  scale_factor=-1  dbl_ovrd=off  block_type=scale
  dout : Outport
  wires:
  din/1 -> debus/1(bus_in)
  debus/1(msb_out16) -> scale1/1
  debus/2(out15) -> scale2/1
  debus/3(out14) -> scale3/1
  debus/4(out13) -> scale4/1
  debus/5(out12) -> scale5/1
  debus/6(out11) -> scale6/1
  debus/7(out10) -> scale7/1
  debus/8(out9) -> scale8/1
  debus/9(out8) -> scale9/1
  debus/10(out7) -> scale10/1
  debus/11(out6) -> scale11/1
  debus/12(out5) -> scale12/1
  debus/13(out4) -> scale13/1
  debus/14(out3) -> scale14/1
  debus/15(out2) -> scale15/1
  debus/16(lsb_out1) -> scale16/1
  scale1/1 -> bussify/1(in1)
  scale2/1 -> bussify/2(in2)
  scale3/1 -> bussify/3(in3)
  scale4/1 -> bussify/4(in4)
  scale5/1 -> bussify/5(in5)
  scale6/1 -> bussify/6(in6)
  scale7/1 -> bussify/7(in7)
  scale8/1 -> bussify/8(in8)
  scale9/1 -> bussify/9(in9)
  scale10/1 -> bussify/10(in10)
  scale11/1 -> bussify/11(in11)
  scale12/1 -> bussify/12(in12)
  scale13/1 -> bussify/13(in13)
  scale14/1 -> bussify/14(in14)
  scale15/1 -> bussify/15(in15)
  scale16/1 -> bussify/16(in16)
  bussify/1(bus_out) -> dout/1

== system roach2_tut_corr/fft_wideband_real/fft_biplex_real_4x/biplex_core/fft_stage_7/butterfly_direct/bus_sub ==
  a : Inport
  b : Inport  Port=2
  a_debus : Subsystem  AncestorBlock=casper_library_flow_control/bus_expand
  addsub{1..8} (8 alike) : xbsIndex_r4/AddSub  mode=Subtraction  use_carryin=off  use_carryout=off  en=off  latency=1  precision=User Defined  arith_type="Signed  (2's comp)"  n_bits=20  bin_pt=17  quantization=Truncate  overflow=Wrap  dbl_ovrd=off  use_behavioral_HDL=on  hw_selection=Fabric  pipelined=on  block_type=addsub
  b_debus : Subsystem  AncestorBlock=casper_library_flow_control/bus_expand
  op_bussify : Subsystem  AncestorBlock=casper_library_flow_control/bus_create
  dout : Outport
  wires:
  a/1 -> a_debus/1(bus_in)
  b/1 -> b_debus/1(bus_in)
  a_debus/1(msb_out8) -> addsub1/1
  b_debus/1(msb_out8) -> addsub1/2
  a_debus/2(out7) -> addsub2/1
  b_debus/2(out7) -> addsub2/2
  a_debus/3(out6) -> addsub3/1
  b_debus/3(out6) -> addsub3/2
  a_debus/4(out5) -> addsub4/1
  b_debus/4(out5) -> addsub4/2
  a_debus/5(out4) -> addsub5/1
  b_debus/5(out4) -> addsub5/2
  a_debus/6(out3) -> addsub6/1
  b_debus/6(out3) -> addsub6/2
  a_debus/7(out2) -> addsub7/1
  b_debus/7(out2) -> addsub7/2
  a_debus/8(lsb_out1) -> addsub8/1
  b_debus/8(lsb_out1) -> addsub8/2
  addsub1/1 -> op_bussify/1(in1)
  addsub2/1 -> op_bussify/2(in2)
  addsub3/1 -> op_bussify/3(in3)
  addsub4/1 -> op_bussify/4(in4)
  addsub5/1 -> op_bussify/5(in5)
  addsub6/1 -> op_bussify/6(in6)
  addsub7/1 -> op_bussify/7(in7)
  addsub8/1 -> op_bussify/8(in8)
  op_bussify/1(bus_out) -> dout/1

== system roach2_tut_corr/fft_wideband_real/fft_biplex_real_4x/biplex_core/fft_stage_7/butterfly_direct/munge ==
  din : Inport
  join : Subsystem  AncestorBlock=casper_library_flow_control/bus_create
  reinterpret : xbsIndex_r4/Reinterpret  force_arith_type=on  arith_type=Unsigned  force_bin_pt=on  bin_pt=0  block_type=reinterpret
  reinterpret_out : xbsIndex_r4/Reinterpret  force_arith_type=on  arith_type=Unsigned  force_bin_pt=on  bin_pt=0  block_type=reinterpret
  split : Subsystem  AncestorBlock=casper_library_flow_control/bus_expand
  dout : Outport
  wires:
  reinterpret_out/1 -> dout/1
  din/1 -> reinterpret/1
  reinterpret/1 -> split/1(bus_in)
  join/1(bus_out) -> reinterpret_out/1
  split/1(msb_out8) -> join/1(in1)
  split/5(out4) -> join/2(in2)
  split/2(out7) -> join/3(in3)
  split/6(out3) -> join/4(in4)
  split/3(out6) -> join/5(in5)
  split/7(out2) -> join/6(in6)
  split/4(out5) -> join/7(in7)
  split/8(lsb_out1) -> join/8(in8)

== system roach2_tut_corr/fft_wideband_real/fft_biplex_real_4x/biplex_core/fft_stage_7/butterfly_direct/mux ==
  sel : Inport
  d0 : Inport  Port=2
  d1 : Inport  Port=3
  d_bussify : Subsystem  AncestorBlock=casper_library_flow_control/bus_create
  expand0 : Subsystem  AncestorBlock=casper_library_flow_control/bus_expand
  expand1 : Subsystem  AncestorBlock=casper_library_flow_control/bus_expand
  mux{0..15} (16 alike) : xbsIndex_r4/Mux  inputs=2  en=off  latency=2  precision=Full  arith_type=Unsigned  n_bits=16  bin_pt=14  quantization=Truncate  overflow=Wrap  dbl_ovrd=off  block_type=mux
  sel_expand : Subsystem  AncestorBlock=casper_library_flow_control/bus_expand
  out : Outport
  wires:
  sel/1 -> sel_expand/1(bus_in)
  d0/1 -> expand0/1(bus_in)
  d1/1 -> expand1/1(bus_in)
  sel_expand/1(msb_out16) -> mux0/1
  expand0/1(msb_out16) -> mux0/2
  expand1/1(msb_out16) -> mux0/3
  sel_expand/2(out15) -> mux1/1
  expand0/2(out15) -> mux1/2
  expand1/2(out15) -> mux1/3
  sel_expand/3(out14) -> mux2/1
  expand0/3(out14) -> mux2/2
  expand1/3(out14) -> mux2/3
  sel_expand/4(out13) -> mux3/1
  expand0/4(out13) -> mux3/2
  expand1/4(out13) -> mux3/3
  sel_expand/5(out12) -> mux4/1
  expand0/5(out12) -> mux4/2
  expand1/5(out12) -> mux4/3
  sel_expand/6(out11) -> mux5/1
  expand0/6(out11) -> mux5/2
  expand1/6(out11) -> mux5/3
  sel_expand/7(out10) -> mux6/1
  expand0/7(out10) -> mux6/2
  expand1/7(out10) -> mux6/3
  sel_expand/8(out9) -> mux7/1
  expand0/8(out9) -> mux7/2
  expand1/8(out9) -> mux7/3
  sel_expand/9(out8) -> mux8/1
  expand0/9(out8) -> mux8/2
  expand1/9(out8) -> mux8/3
  sel_expand/10(out7) -> mux9/1
  expand0/10(out7) -> mux9/2
  expand1/10(out7) -> mux9/3
  sel_expand/11(out6) -> mux10/1
  expand0/11(out6) -> mux10/2
  expand1/11(out6) -> mux10/3
  sel_expand/12(out5) -> mux11/1
  expand0/12(out5) -> mux11/2
  expand1/12(out5) -> mux11/3
  sel_expand/13(out4) -> mux12/1
  expand0/13(out4) -> mux12/2
  expand1/13(out4) -> mux12/3
  sel_expand/14(out3) -> mux13/1
  expand0/14(out3) -> mux13/2
  expand1/14(out3) -> mux13/3
  sel_expand/15(out2) -> mux14/1
  expand0/15(out2) -> mux14/2
  expand1/15(out2) -> mux14/3
  sel_expand/16(lsb_out1) -> mux15/1
  expand0/16(lsb_out1) -> mux15/2
  expand1/16(lsb_out1) -> mux15/3
  mux0/1 -> d_bussify/1(in1)
  mux1/1 -> d_bussify/2(in2)
  mux2/1 -> d_bussify/3(in3)
  mux3/1 -> d_bussify/4(in4)
  mux4/1 -> d_bussify/5(in5)
  mux5/1 -> d_bussify/6(in6)
  mux6/1 -> d_bussify/7(in7)
  mux7/1 -> d_bussify/8(in8)
  mux8/1 -> d_bussify/9(in9)
  mux9/1 -> d_bussify/10(in10)
  mux10/1 -> d_bussify/11(in11)
  mux11/1 -> d_bussify/12(in12)
  mux12/1 -> d_bussify/13(in13)
  mux13/1 -> d_bussify/14(in14)
  mux14/1 -> d_bussify/15(in15)
  mux15/1 -> d_bussify/16(in16)
  d_bussify/1(bus_out) -> out/1

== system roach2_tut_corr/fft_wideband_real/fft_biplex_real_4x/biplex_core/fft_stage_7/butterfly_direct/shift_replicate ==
  in : Inport
  bussify : Subsystem  AncestorBlock=casper_library_flow_control/bus_create
  din0_{0..15} (16 alike) : xbsIndex_r4/Delay  rst=off  infoeditControl=Selection of Reset will increase slice count due to use of real FFs and instead of SRLs  en=off  latency=1  dbl_ovrd=off  reg_retiming=off  block_type=delay
  out : Outport
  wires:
  in/1 -> din0_0/1, din0_1/1, din0_2/1, din0_3/1, din0_4/1, din0_5/1, din0_6/1, din0_7/1, din0_8/1, din0_9/1, din0_10/1, din0_11/1, din0_12/1, din0_13/1, din0_14/1, din0_15/1
  din0_0/1 -> bussify/1(in1)
  din0_1/1 -> bussify/2(in2)
  din0_2/1 -> bussify/3(in3)
  din0_3/1 -> bussify/4(in4)
  din0_4/1 -> bussify/5(in5)
  din0_5/1 -> bussify/6(in6)
  din0_6/1 -> bussify/7(in7)
  din0_7/1 -> bussify/8(in8)
  din0_8/1 -> bussify/9(in9)
  din0_9/1 -> bussify/10(in10)
  din0_10/1 -> bussify/11(in11)
  din0_11/1 -> bussify/12(in12)
  din0_12/1 -> bussify/13(in13)
  din0_13/1 -> bussify/14(in14)
  din0_14/1 -> bussify/15(in15)
  din0_15/1 -> bussify/16(in16)
  bussify/1(bus_out) -> out/1

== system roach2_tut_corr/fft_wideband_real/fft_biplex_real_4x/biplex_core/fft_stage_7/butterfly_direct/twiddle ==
  ai : Inport
  bi : Inport  Port=2
  sync_in : Inport  Port=3
  bus_convert : Subsystem  AncestorBlock=casper_library_bus/bus_convert
  bus_create : Subsystem  AncestorBlock=casper_library_flow_control/bus_create
  bus_expand : Subsystem  AncestorBlock=casper_library_flow_control/bus_expand
  bus_expand1 : Subsystem  AncestorBlock=casper_library_flow_control/bus_expand
  bus_mult : Subsystem  AncestorBlock=casper_library_bus/bus_mult
  coeff_gen : Subsystem  AncestorBlock=casper_library_ffts_twiddle_coeff_gen/coeff_gen
  ao : Outport
  bwo : Outport  Port=2
  sync_out : Outport  Port=3
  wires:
  bi/1 -> bus_create/1(in1)
  sync_in/1 -> bus_create/2(in2), coeff_gen/1(rst)
  ai/1 -> bus_create/3(in3)
  bus_create/1(bus_out) -> coeff_gen/2(misci)
  coeff_gen/2(misco) -> bus_expand/1(bus_in)
  coeff_gen/1(w) -> bus_mult/1(a)
  bus_expand/2(lsb_out1) -> bus_mult/3(misci)
  bus_expand/1(msb_out2) -> bus_mult/2(b)
  bus_mult/1(a*b) -> bus_convert/1(din)
  bus_mult/2(misco) -> bus_convert/2(misci)
  bus_convert/1(dout) -> bwo/1
  bus_convert/2(misco) -> bus_expand1/1(bus_in)
  bus_expand1/1(msb_out2) -> sync_out/1
  bus_expand1/2(lsb_out1) -> ao/1

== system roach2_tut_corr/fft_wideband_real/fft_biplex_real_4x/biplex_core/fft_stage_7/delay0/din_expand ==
  bus_in : Inport
  reinterpret{1..4} (4 alike) : xbsIndex_r4/Reinterpret  force_arith_type=on  arith_type=Unsigned  force_bin_pt=on  bin_pt=0  block_type=reinterpret
  slice1 : xbsIndex_r4/Slice  nbits=36  boolean_output=off  mode=Upper Bit Location + Width  bit1=-108  base1=MSB of Input  bit0=0  base0=LSB of Input  dbl_ovrd=off  block_type=slice
  slice2 : xbsIndex_r4/Slice  nbits=36  boolean_output=off  mode=Upper Bit Location + Width  bit1=-72  base1=MSB of Input  bit0=0  base0=LSB of Input  dbl_ovrd=off  block_type=slice
  slice3 : xbsIndex_r4/Slice  nbits=36  boolean_output=off  mode=Upper Bit Location + Width  bit1=-36  base1=MSB of Input  bit0=0  base0=LSB of Input  dbl_ovrd=off  block_type=slice
  slice4 : xbsIndex_r4/Slice  nbits=36  boolean_output=off  mode=Upper Bit Location + Width  bit1=0  base1=MSB of Input  bit0=0  base0=LSB of Input  dbl_ovrd=off  block_type=slice
  msb_out4 : Outport
  out3 : Outport  Port=2
  out2 : Outport  Port=3
  lsb_out1 : Outport  Port=4
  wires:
  bus_in/1 -> slice4/1, slice3/1, slice2/1, slice1/1
  slice4/1 -> reinterpret4/1
  reinterpret4/1 -> msb_out4/1
  slice3/1 -> reinterpret3/1
  reinterpret3/1 -> out3/1
  slice2/1 -> reinterpret2/1
  reinterpret2/1 -> out2/1
  slice1/1 -> reinterpret1/1
  reinterpret1/1 -> lsb_out1/1

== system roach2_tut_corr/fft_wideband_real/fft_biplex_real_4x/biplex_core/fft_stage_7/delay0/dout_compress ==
  in1 : Inport
  in2 : Inport  Port=2
  in3 : Inport  Port=3
  in4 : Inport  Port=4
  concatenate : xbsIndex_r4/Concat  num_inputs=4  dbl_ovrd=off  block_type=concat
  reinterpret{1..4} (4 alike) : xbsIndex_r4/Reinterpret  force_arith_type=on  arith_type=Unsigned  force_bin_pt=on  bin_pt=0  block_type=reinterpret
  bus_out : Outport
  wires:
  concatenate/1 -> bus_out/1
  in1/1 -> reinterpret1/1
  reinterpret1/1 -> concatenate/1
  in2/1 -> reinterpret2/1
  reinterpret2/1 -> concatenate/2
  in3/1 -> reinterpret3/1
  reinterpret3/1 -> concatenate/3
  in4/1 -> reinterpret4/1
  reinterpret4/1 -> concatenate/4

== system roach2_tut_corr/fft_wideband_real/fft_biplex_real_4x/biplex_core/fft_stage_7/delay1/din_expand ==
  bus_in : Inport
  reinterpret{1..4} (4 alike) : xbsIndex_r4/Reinterpret  force_arith_type=on  arith_type=Unsigned  force_bin_pt=on  bin_pt=0  block_type=reinterpret
  slice1 : xbsIndex_r4/Slice  nbits=36  boolean_output=off  mode=Upper Bit Location + Width  bit1=-108  base1=MSB of Input  bit0=0  base0=LSB of Input  dbl_ovrd=off  block_type=slice
  slice2 : xbsIndex_r4/Slice  nbits=36  boolean_output=off  mode=Upper Bit Location + Width  bit1=-72  base1=MSB of Input  bit0=0  base0=LSB of Input  dbl_ovrd=off  block_type=slice
  slice3 : xbsIndex_r4/Slice  nbits=36  boolean_output=off  mode=Upper Bit Location + Width  bit1=-36  base1=MSB of Input  bit0=0  base0=LSB of Input  dbl_ovrd=off  block_type=slice
  slice4 : xbsIndex_r4/Slice  nbits=36  boolean_output=off  mode=Upper Bit Location + Width  bit1=0  base1=MSB of Input  bit0=0  base0=LSB of Input  dbl_ovrd=off  block_type=slice
  msb_out4 : Outport
  out3 : Outport  Port=2
  out2 : Outport  Port=3
  lsb_out1 : Outport  Port=4
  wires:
  bus_in/1 -> slice4/1, slice3/1, slice2/1, slice1/1
  slice4/1 -> reinterpret4/1
  reinterpret4/1 -> msb_out4/1
  slice3/1 -> reinterpret3/1
  reinterpret3/1 -> out3/1
  slice2/1 -> reinterpret2/1
  reinterpret2/1 -> out2/1
  slice1/1 -> reinterpret1/1
  reinterpret1/1 -> lsb_out1/1

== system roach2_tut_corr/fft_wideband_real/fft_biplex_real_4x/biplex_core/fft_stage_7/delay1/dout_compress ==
  in1 : Inport
  in2 : Inport  Port=2
  in3 : Inport  Port=3
  in4 : Inport  Port=4
  concatenate : xbsIndex_r4/Concat  num_inputs=4  dbl_ovrd=off  block_type=concat
  reinterpret{1..4} (4 alike) : xbsIndex_r4/Reinterpret  force_arith_type=on  arith_type=Unsigned  force_bin_pt=on  bin_pt=0  block_type=reinterpret
  bus_out : Outport
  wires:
  concatenate/1 -> bus_out/1
  in1/1 -> reinterpret1/1
  reinterpret1/1 -> concatenate/1
  in2/1 -> reinterpret2/1
  reinterpret2/1 -> concatenate/2
  in3/1 -> reinterpret3/1
  reinterpret3/1 -> concatenate/3
  in4/1 -> reinterpret4/1
  reinterpret4/1 -> concatenate/4

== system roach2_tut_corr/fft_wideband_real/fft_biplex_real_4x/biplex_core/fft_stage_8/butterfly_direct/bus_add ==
  a : Inport
  b : Inport  Port=2
  a_debus : Subsystem  AncestorBlock=casper_library_flow_control/bus_expand
  addsub{1..8} (8 alike) : xbsIndex_r4/AddSub  mode=Addition  use_carryin=off  use_carryout=off  en=off  latency=1  precision=User Defined  arith_type="Signed  (2's comp)"  n_bits=20  bin_pt=17  quantization=Truncate  overflow=Wrap  dbl_ovrd=off  use_behavioral_HDL=on  hw_selection=Fabric  pipelined=on  block_type=addsub
  b_debus : Subsystem  AncestorBlock=casper_library_flow_control/bus_expand
  op_bussify : Subsystem  AncestorBlock=casper_library_flow_control/bus_create
  dout : Outport
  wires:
  a/1 -> a_debus/1(bus_in)
  b/1 -> b_debus/1(bus_in)
  a_debus/1(msb_out8) -> addsub1/1
  b_debus/1(msb_out8) -> addsub1/2
  a_debus/2(out7) -> addsub2/1
  b_debus/2(out7) -> addsub2/2
  a_debus/3(out6) -> addsub3/1
  b_debus/3(out6) -> addsub3/2
  a_debus/4(out5) -> addsub4/1
  b_debus/4(out5) -> addsub4/2
  a_debus/5(out4) -> addsub5/1
  b_debus/5(out4) -> addsub5/2
  a_debus/6(out3) -> addsub6/1
  b_debus/6(out3) -> addsub6/2
  a_debus/7(out2) -> addsub7/1
  b_debus/7(out2) -> addsub7/2
  a_debus/8(lsb_out1) -> addsub8/1
  b_debus/8(lsb_out1) -> addsub8/2
  addsub1/1 -> op_bussify/1(in1)
  addsub2/1 -> op_bussify/2(in2)
  addsub3/1 -> op_bussify/3(in3)
  addsub4/1 -> op_bussify/4(in4)
  addsub5/1 -> op_bussify/5(in5)
  addsub6/1 -> op_bussify/6(in6)
  addsub7/1 -> op_bussify/7(in7)
  addsub8/1 -> op_bussify/8(in8)
  op_bussify/1(bus_out) -> dout/1
